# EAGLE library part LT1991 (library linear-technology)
Precision 100μA Gain Selectable Amplifier Data sheet
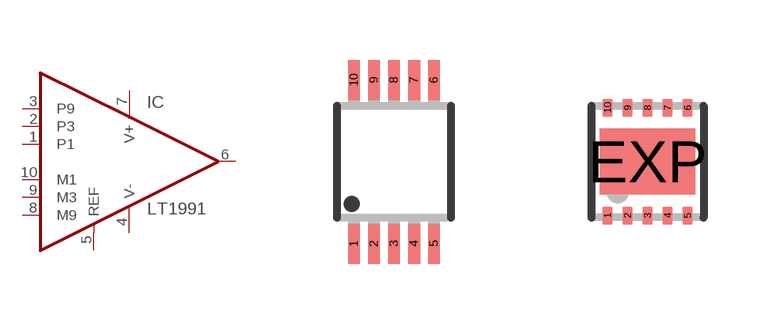
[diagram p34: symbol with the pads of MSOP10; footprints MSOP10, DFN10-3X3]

Designator prefix IC

## LT1991MS  [MSOP10]
1  P1  in
2  P3  in
3  P9  in
4  V-  pwr
5  REF  in
6  OUT  out
7  V+  pwr
8  M9  in
9  M3  in
10  M1  in

## LT1991DD  [DFN10-3X3]
1  P1  in
2  P3  in
3  P9  in
4  V-  pwr
5  REF  in
6  OUT  out
7  V+  pwr
8  M9  in
9  M3  in
10  M1  in
EXP  V-  pwr

## Footprint MSOP10 (pad centres in mm)
10 Lead Platic MSOP Source: http://www.linear.com .. LT1996
smd 0.3 x 1: 1 -1,-2.05; 2 -0.5,-2.05; 3 0,-2.05; 4 0.5,-2.05; 5 1,-2.05; 6 1,2.05; 7 0.5,2.05; 8 0,2.05; 9 -0.5,2.05; 10 -1,2.05

## Footprint DFN10-3X3 (pad centres in mm)
DD Package 10-Lead Plastic DFN (3mm × 3mm) (Reference LTC DWG # 05-08-1669) Source: http://www.linear.com .. 4062fa.pdf
smd 0.25 x 0.45: 1 -1,-1.35; 2 -0.5,-1.35; 3 0,-1.35; 4 0.5,-1.35; 5 1,-1.35; 6 1,1.35; 7 0.5,1.35; 8 0,1.35; 9 -0.5,1.35; 10 -1,1.35
smd 2.38 x 1.65: EXP 0,0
